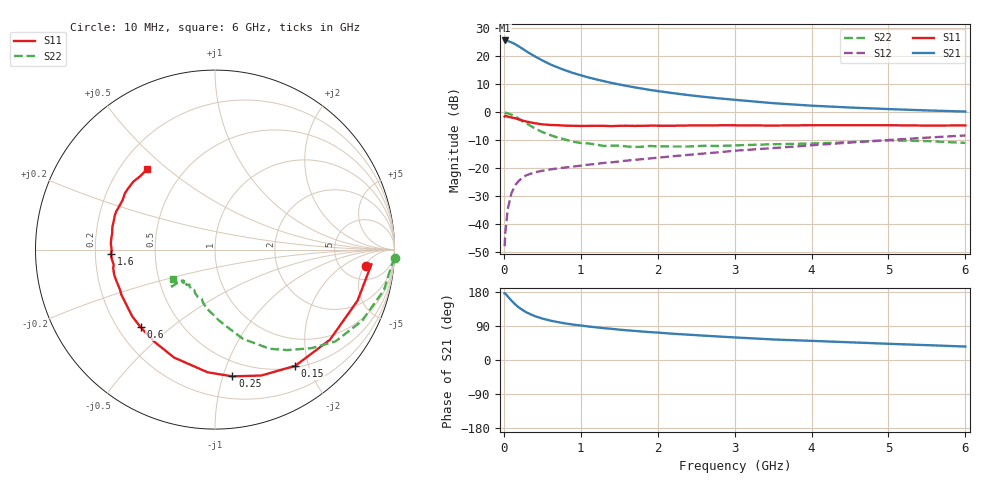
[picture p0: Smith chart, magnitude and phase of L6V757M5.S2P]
!  INFINEON TECHNOLOGIES Small Signal Semiconductors
! BFR380L3 , Si-NPN RF-Transistor in TSLP-3-1
!  Vce=0.75 V,  Ic=7.5 mA
! Common Emitter S-Parameters:  07. March 2005
#  GHz  S  MA  R  50
! f  S11  S21  S12  S22
! GHz  Mag  Ang  Mag  Ang  Mag  Ang  Mag  Ang
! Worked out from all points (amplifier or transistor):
!   36 points, 10 MHz to 6 GHz, reference 50 ohm
!   highest |S21| = 25.7 dB at 10 MHz (marker M1)
!   |S21| within 3 dB of that: start of sweep to 245.5 MHz
!   unconditionally stable (mu >= 1): 2.103 GHz to 5.02 GHz
!   at 250 MHz: K = 0.23, MSG = 22.9 dB, |S12| = -23.1 dB
!   at 1.4 GHz: K = 0.87, MSG = 14.2 dB, |S12| = -17.8 dB
!   at 6 GHz: K = 0.99, MSG = 4.3 dB, |S12| = -8.2 dB
!   S11 on the Smith chart (normalised r, x): 10 MHz: 8.25, -5.39; 150 MHz: 0.53, -1.79; 250 MHz: 0.37, -1.07; 600 MHz: 0.29, -0.40; 1.6 GHz: 0.27, -0.02; 6 GHz: 0.31, +0.43
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0.01  0.8438 -6.4  19.32 175.9  0.0041 81.7  1.004 -2.7
0.02  0.8758 -5.3  19.24 175.4  0.0072 88.6  0.9857 -5.5
0.05  0.8436 -19.7  18.93 167.8  0.0186 80.8  0.9682 -13.4
0.1  0.8137 -38.1  17.82 156.6  0.0365 71.6  0.9105 -25.8
0.15  0.7868 -55.4  16.52 146.3  0.0508 63.0  0.8438 -37.3
0.2  0.7475 -69.8  14.97 137.9  0.0613 57.5  0.7667 -45.8
0.25  0.7129 -82.2  13.55 131.1  0.0697 52.5  0.6885 -54.4
0.3  0.6847 -93.5  12.2 125.0  0.0763 49.3  0.6311 -61.1
0.4  0.6432 -110.8  10.11 115.9  0.0852 44.5  0.5222 -72.5
0.5  0.6143 -123.5  8.512 109.4  0.091 42.6  0.4474 -79.7
0.6  0.5991 -133.8  7.272 104.1  0.0958 41.1  0.3962 -86.7
0.8  0.5815 -148.1  5.657 96.5  0.1042 41.3  0.3281 -98.7
0.9  0.5791 -154.1  5.068 93.5  0.1079 41.7  0.2999 -103.2
1.1  0.5764 -162.0  4.224 88.4  0.117 43.4  0.2807 -109.9
1.4  0.5708 -171.6  3.369 82.3  0.1287 45.9  0.2556 -117.8
1.6  0.5805 -177.7  2.976 78.3  0.1383 47.3  0.2472 -125.4
2.2  0.5801 170.8  2.213 69.3  0.1656 51.4  0.2468 -130.5
2.8  0.5897 161.1  1.784 61.9  0.1951 54.5  0.2522 -137.0
3.5  0.5838 152.0  1.466 54.2  0.2313 55.3  0.2711 -137.9
4.5  0.5919 144.6  1.226 46.7  0.2905 56.6  0.2958 -139.0
5.5  0.5836 135.3  1.088 39.2  0.3551 54.7  0.3087 -140.9
6  0.5868 129.9  1.039 35.5  0.3891 53.2  0.2859 -144.4
